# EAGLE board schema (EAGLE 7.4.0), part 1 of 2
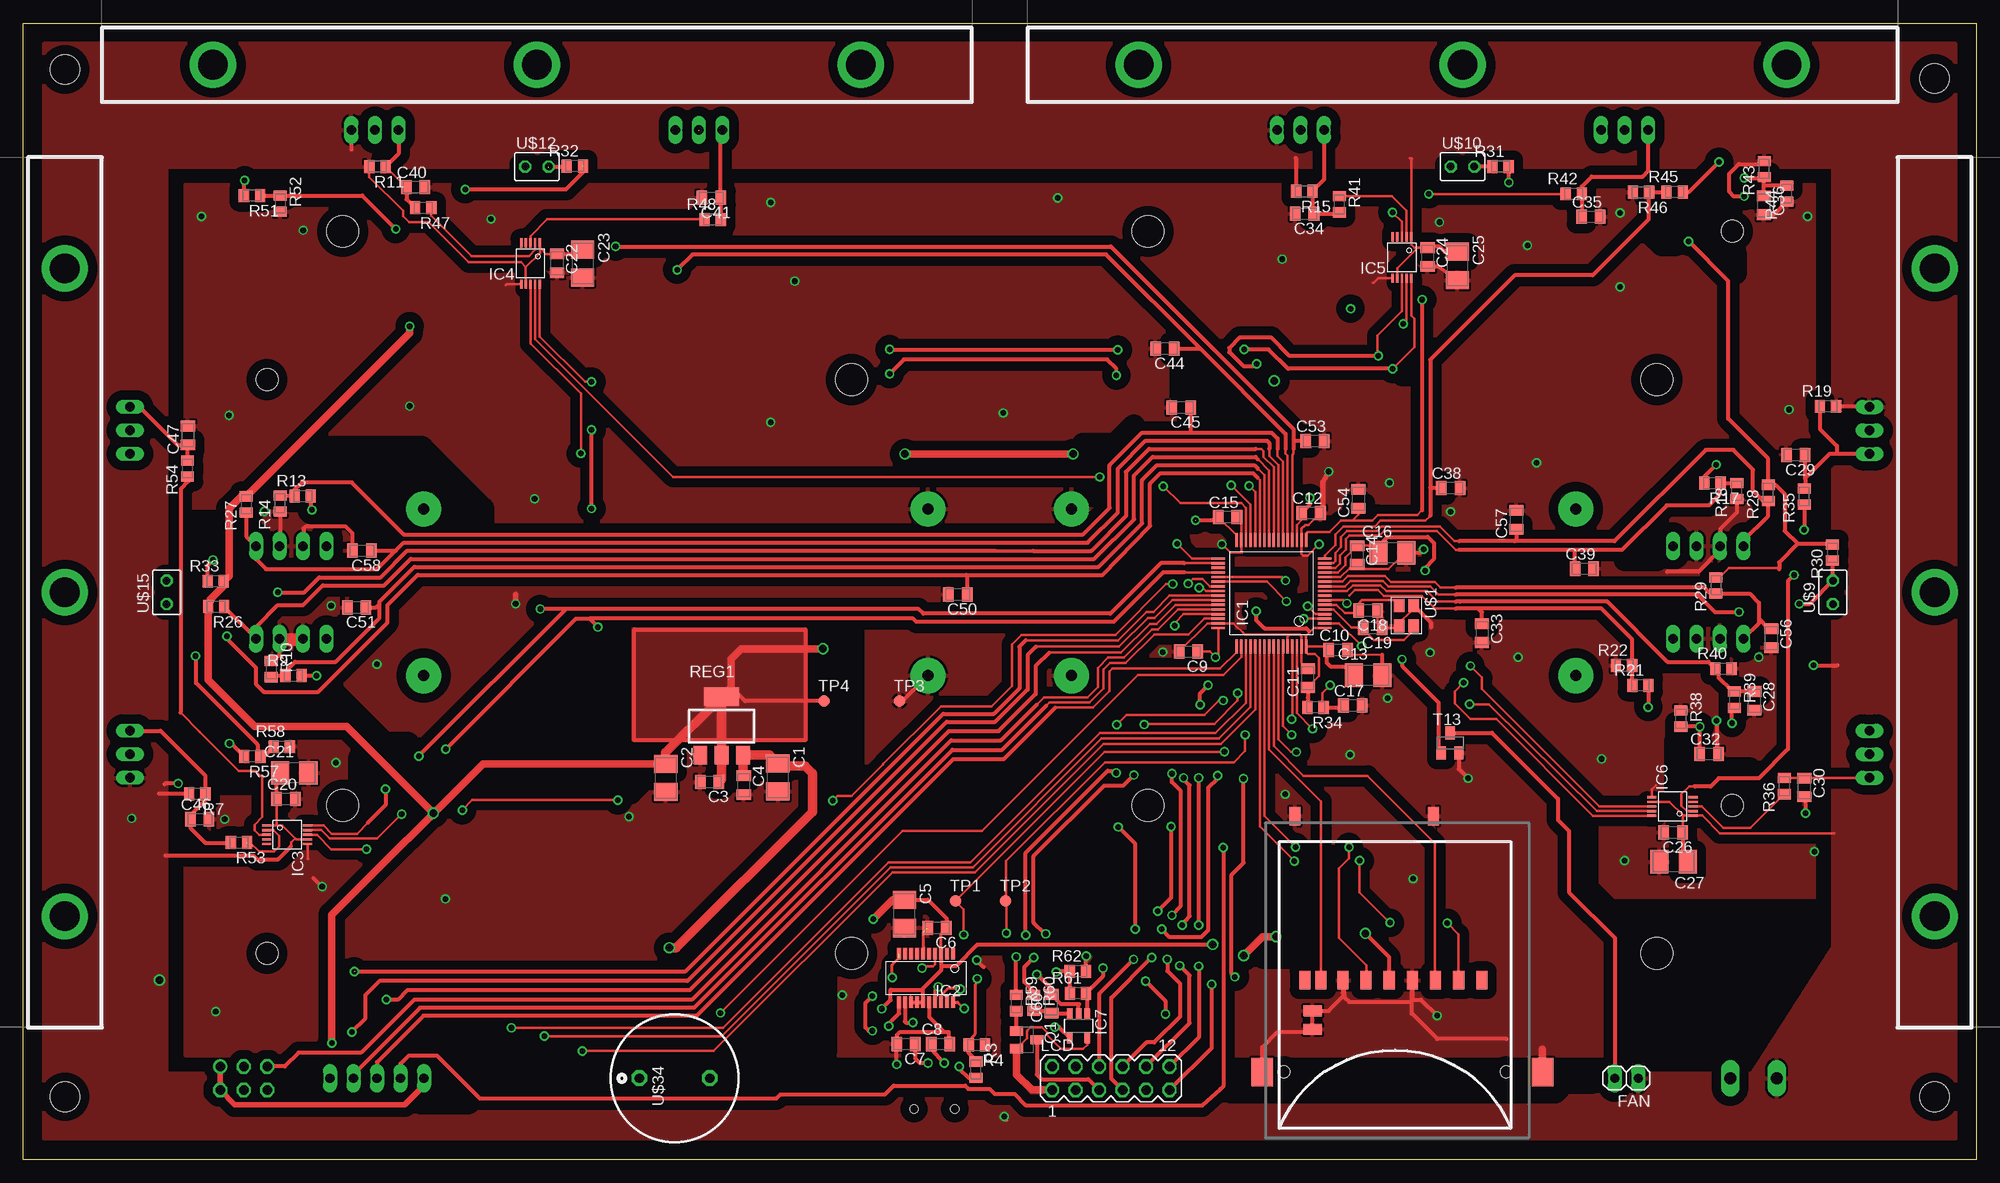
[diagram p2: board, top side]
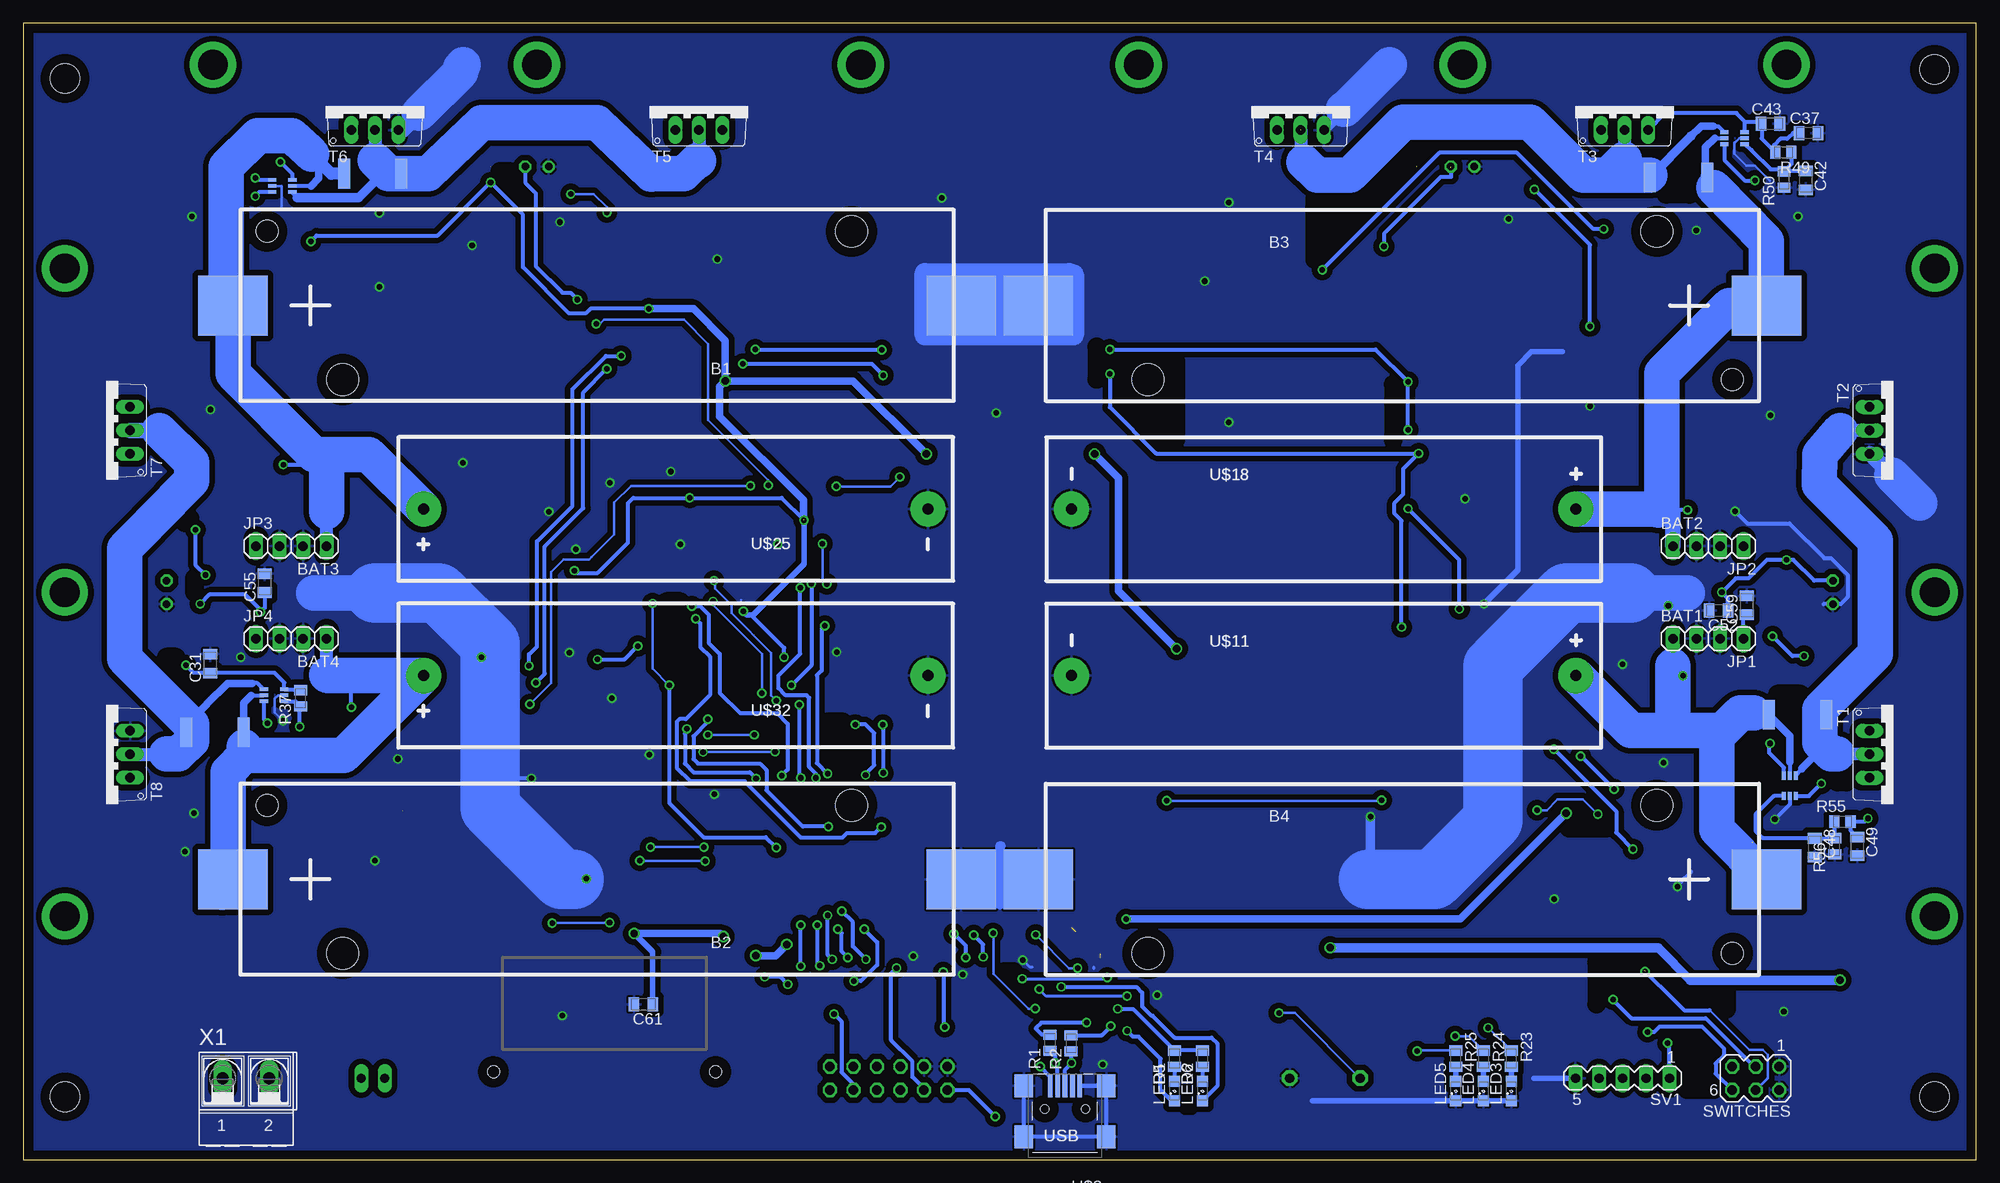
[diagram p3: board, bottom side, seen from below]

Size 211 x 122.79 mm. Coordinates in mm from the lower left corner, seen from the top.
Outline: 0,0 0,122.79 211,122.79 211,0 0,0
Copper layers (1*16): Top 0.035mm / dielectric 1.5mm / Bottom 0.035mm
Design rules "default2": minimum track width 10mil, minimum drill 0.6mm, track to track 8mil, track to pad 8mil, pad to pad 8mil, via to via 8mil, smd to smd 8mil, copper to edge 40mil, drill to drill 8mil, minimum pad ring 10mil, minimum via ring 8mil, stop-mask expansion 4mil, vias tented up to drill 0mil, thermal gap 10mil
Holes 3.2 mm at 4.5,6.79 206.5,6.79 206.5,116.79 4.5,117.79
tRestrict: area 172.2,26.2 to 193.6,27.1; 45 lines
bRestrict: area 51.2,7 to 52.1,7.4; area 54.4,7.2 to 55,7.4; area 84.8,5.4 to 85.5,5.7; area 177.1,110.5 to 177.8,110.7; 19 lines

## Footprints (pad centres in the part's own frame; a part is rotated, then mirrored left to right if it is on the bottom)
KEYSTONE1042 = smd 7.493 x 6.477: P$1 -39.332,0; P$2 39.332,0 | hole 3.454: -27.495,-8.001; 27.495,8.001 | hole 2.388: 35.662,-8.001
1X02 = drill 1.016 long: 1 -1.27,0; 2 1.27,0
SMDB = smd 1.95 x 2.5: P$1 -1.525,0; P$2 1.525,0
SMD0805C = smd 1.143 x 1.524: P$1 -1.016,0; P$2 1.016,0
LQFP64 = smd 0.254 x 1.5: P$1 -3.75,-5.75; P$2 -3.25,-5.75; P$3 -2.75,-5.75; P$4 -2.25,-5.75; P$5 -1.75,-5.75; P$6 -1.25,-5.75; P$7 -0.75,-5.75; P$8 -0.25,-5.75; P$9 0.25,-5.75; P$10 0.75,-5.75; P$11 1.25,-5.75; P$12 1.75,-5.75; P$13 2.25,-5.75; P$14 2.75,-5.75; P$15 3.25,-5.75; P$16 3.75,-5.75; P$33 3.75,5.75; P$34 3.25,5.75; P$35 2.75,5.75; P$36 2.25,5.75; P$37 1.75,5.75; P$38 1.25,5.75; P$39 0.75,5.75; P$40 0.25,5.75; P$41 -0.25,5.75; P$42 -0.75,5.75; P$43 -1.25,5.75; P$44 -1.75,5.75; P$45 -2.25,5.75; P$46 -2.75,5.75; P$47 -3.25,5.75; P$48 -3.75,5.75 | smd 1.5 x 0.254: P$17 5.75,-3.75; P$18 5.75,-3.25; P$19 5.75,-2.75; P$20 5.75,-2.25; P$21 5.75,-1.75; P$22 5.75,-1.25; P$23 5.75,-0.75; P$24 5.75,-0.25; P$25 5.75,0.25; P$26 5.75,0.75; P$27 5.75,1.25; P$28 5.75,1.75; P$29 5.75,2.25; P$30 5.75,2.75; P$31 5.75,3.25; P$32 5.75,3.75; P$49 -5.75,3.75; P$50 -5.75,3.25; P$51 -5.75,2.75; P$52 -5.75,2.25; P$53 -5.75,1.75; P$54 -5.75,1.25; P$55 -5.75,0.75; P$56 -5.75,0.25; P$57 -5.75,-0.25; P$58 -5.75,-0.75; P$59 -5.75,-1.25; P$60 -5.75,-1.75; P$61 -5.75,-2.25; P$62 -5.75,-2.75; P$63 -5.75,-3.25; P$64 -5.75,-3.75
SSOP20 = smd 0.42 x 1.25: P$1 -2.925,-2.625; P$2 -2.275,-2.625; P$3 -1.625,-2.625; P$4 -0.975,-2.625; P$5 -0.325,-2.625; P$6 0.325,-2.625; P$7 0.975,-2.625; P$8 1.625,-2.625; P$9 2.275,-2.625; P$10 2.925,-2.625; P$11 2.925,2.625; P$12 2.275,2.625; P$13 1.625,2.625; P$14 0.975,2.625; P$15 0.325,2.625; P$16 -0.325,2.625; P$17 -0.975,2.625; P$18 -1.625,2.625; P$19 -2.275,2.625; P$20 -2.925,2.625
VSSOP = smd 0.254 x 1: P$1 -1,-2.225; P$2 -0.5,-2.225; P$3 0,-2.225; P$4 0.5,-2.225; P$5 1,-2.225; P$6 1,2.225; P$7 0.5,2.225; P$8 0,2.225; P$9 -0.5,2.225; P$10 -1,2.225
SOT23-5 = smd 0.6 x 1.2: 1 -0.95,-1.306; 2 0,-1.306; 3 0.95,-1.306; 4 0.95,1.306; 5 -0.95,1.306
MA06-2 = drill 1.016 octagon: 1 -6.35,-1.27; 2 -6.35,1.27; 3 -3.81,-1.27; 4 -3.81,1.27; 5 -1.27,-1.27; 6 -1.27,1.27; 7 1.27,-1.27; 8 1.27,1.27; 9 3.81,-1.27; 10 3.81,1.27; 11 6.35,-1.27; 12 6.35,1.27
SML0805 = smd 1.2 x 1.2: A 1.05,0; C -1.05,0
SOT23-BEC = smd 1 x 1.4: B -0.95,-1.1; C 0,1.1; E 0.95,-1.1
SMD0805R = smd 1.1 x 1.4: P$1 -0.875,0; P$2 0.875,0
CURRENT_SENSE = smd 1.3 x 3.2: P$1 -3.1,0; P$2 3.1,0
SOT223 = smd 1.5 x 2: P$1 -2.3,-3.15; P$2 0,-3.15; P$3 2.3,-3.15 | smd 3.8 x 2: P$4 0,3.15
MA05-1 = drill 1.016 long: 1 -5.08,0; 2 -2.54,0; 3 0,0; 4 2.54,0; 5 5.08,0
MA03-2 = drill 1.016: 1 -2.54,-1.27 | drill 1.016 octagon: 2 -2.54,1.27; 3 0,-1.27; 4 0,1.27; 5 2.54,-1.27; 6 2.54,1.27
TO220 = drill 1.016 long: P$1 -2.54,-2.54; P$2 0,-2.54; P$3 2.54,-2.54
SOT23 = smd 1 x 1.4: 1 -0.95,-1.1; 2 0.95,-1.1; 3 0,1.1
B1,27 = smd 1.27 x 1.27: TP 0,0
XTAL-TSX-3225 = smd 1.4 x 1.15: GND1 -1.1,0.8; GND2 1.1,-0.8; P$2 1.1,0.8; P$4 -1.1,-0.8
DCK(INA213) = smd 0.4 x 0.9: P$1 -0.65,-1.1; P$2 0,-1.1; P$3 0.65,-1.1; P$4 0.65,1.1; P$5 0,1.1; P$6 -0.65,1.1
USB-MINI = smd 2 x 2.5: M1 -4.45,-2.25; M2 4.45,-2.25; M3 -4.45,-7.75; M4 4.45,-7.75 | smd 0.5 x 2.5: P$1 1.6,-7.75; P$2 0.8,-7.75; P$3 0,-7.75; P$4 -0.8,-7.75; P$5 -1.6,-7.75 | hole 0.9: -2.2,-5.25; 2.2,-5.25
THERMISTOR = drill 0.813 octagon: 1 -1.27,0; 2 1.27,0
KEYSTONE1015 = drill 1.2 pad 3.81: P$1 -27.241,0; P$2 27.241,0
CHLADIC = drill 3.2 pad 5: P$1 -35,23.5; P$2 0,23.5; P$4 35,23.5
SD-SOCKET = smd 1.2 x 2: DC -10.83,17.75; OPT 4.15,17.75; P$1 6.87,0; P$2 4.37,0; P$3 1.87,0; P$4 -0.63,0; P$5 -3.13,0; P$6 -5.63,0; P$7 -8,0; P$8 -9.75,0; P$9 9.37,0 | smd 2 x 1.2: GND -8.9,-3.3; WP -8.9,-5.3 | smd 2.3 x 3.1: M1 15.95,-9.9; M2 -14.35,-9.9 | hole 1.3: 12,-9.9; -12,-9.9
12N40 = drill 1 pad 1.676 octagon: P$1 0,3.8; P$2 0,-3.8
AK500/2-H = drill 1.321 long: 1 -2.515,0; 2 2.515,0

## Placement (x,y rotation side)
B1  BATTERY-LI  [KEYSTONE1042]  149,92.29 180 bottom
B2  BATTERY-LI  [KEYSTONE1042]  149,30.29 180 bottom
B3  BATTERY-LI  [KEYSTONE1042]  62,92.29 0 bottom
B4  BATTERY-LI  [KEYSTONE1042]  62,30.29 0 bottom
BAT1  [1X02]  31.5,56.29 0 bottom
BAT2  [1X02]  31.5,66.29 0 bottom
BAT3  [1X02]  179.5,66.29 180 bottom
BAT4  [1X02]  179.5,56.29 180 bottom
C1  10uF  [SMDB]  81.53,41.29 270 top
C2  10uF  [SMDB]  69.42,41.24 270 top
C3  100n  [SMD0805C]  74.15,40.81 180 top
C4  100n  [SMD0805C]  77.85,40.46 270 top
C5  4.7uF  [SMDB]  95.2,26.54 270 top
C6  100n  [SMD0805C]  98.72,25.04 180 top
C7  47pF  [SMD0805C]  95.38,12.49 180 top
C8  47pF  [SMD0805C]  99.1,12.49 0 top
C9  100n  [SMD0805C]  125.88,54.88 180 top
C10  100n  [SMD0805C]  142.07,55.06 0 top
C11  100n  [SMD0805C]  138.77,52.02 90 top
C12  100n  [SMD0805C]  139.13,69.87 0 top
C13  10uF  [SMDB]  145.3,52.33 0 top
C14  100n  [SMD0805C]  144.11,65.31 270 top
C15  100n  [SMD0805C]  130.11,69.41 0 top
C16  1uF  [SMDB]  147.91,65.57 0 top
C17  100n  [SMD0805C]  143.64,49.06 0 top
C18  25pF  [SMD0805C]  145.3,59.34 180 top
C19  25pF  [SMD0805C]  145.77,57.44 180 top
C20  100n  [SMD0805C]  28.39,38.96 0 top
C21  10uF  [SMDB]  29.3,41.79 0 top
C22  100n  [SMD0805C]  57.67,96.83 270 top
C23  10uF  [SMDB]  60.45,96.81 270 top
C24  100n  [SMD0805C]  151.72,97.51 270 top
C25  10uF  [SMDB]  154.93,96.55 270 top
C26  100n  [SMD0805C]  178.25,35.34 180 top
C27  10uF  [SMDB]  178.3,32.19 180 top
C28  100n  [SMD0805C]  187,49.56 270 top
C29  22n  [SMD0805C]  191.5,76.11 180 top
C30  22n  [SMD0805C]  192.43,40.21 270 top
C31  100n  [SMD0805C]  190.8,53.59 90 bottom
C32  100n  [SMD0805C]  182.12,43.84 0 top
C33  100n  [SMD0805C]  157.6,56.89 270 top
C34  22n  [SMD0805C]  138.43,102.19 180 top
C35  22n  [SMD0805C]  169.35,101.86 0 top
C36  100n  [SMD0805C]  188.05,103.11 270 top
C37  100n  [SMD0805C]  18.12,110.91 0 bottom
C38  100n  [SMD0805C]  154.2,72.56 0 top
C39  100n  [SMD0805C]  168.65,63.84 0 top
C40  22n  [SMD0805C]  42.4,105.06 0 top
C41  22n  [SMD0805C]  74.35,103.91 180 top
C42  100n  [SMD0805C]  18.42,105.79 270 bottom
C43  100n  [SMD0805C]  22.25,111.91 0 bottom
C44  100n  [SMD0805C]  123.35,87.61 180 top
C45  100n  [SMD0805C]  125.1,81.26 180 top
C46  22n  [SMD0805C]  19.08,36.79 0 top
C47  22n  [SMD0805C]  17.8,78.24 90 top
C48  100n  [SMD0805C]  17.45,33.69 270 bottom
C49  100n  [SMD0805C]  12.88,33.84 270 bottom
C50  100n  [SMD0805C]  100.97,61.06 180 top
C51  100n  [SMD0805C]  36.03,59.66 180 top
C52  100n  [SMD0805C]  27.85,59.34 180 bottom
C53  100n  [SMD0805C]  139.55,77.64 0 top
C54  100n  [SMD0805C]  144.25,71.39 90 top
C55  100n  [SMD0805C]  184.9,62.29 90 bottom
C56  100n  [SMD0805C]  188.85,56.34 270 top
C57  100n  [SMD0805C]  161.3,69.14 90 top
C58  100n  [SMD0805C]  36.6,65.79 180 top
C59  100n  [SMD0805C]  24.8,59.89 90 bottom
C60  100n  [SMD0805C]  111.07,16.84 90 top
C61  100n  [SMD0805C]  144,16.79 180 bottom
FAN  [1X02]  173.21,8.79 180 top
IC1  [LQFP64]  134.85,61.19 90 top
IC2  FT231XS  [SSOP20]  97.53,19.63 180 top
IC3  DAC122S085  [VSSOP]  28.52,35.1 270 top
IC4  DAC122S085  [VSSOP]  54.8,96.81 180 top
IC5  DAC122S085  [VSSOP]  148.94,97.46 180 top
IC6  DAC122S085  [VSSOP]  178.18,38.15 90 top
IC7  MCP601OT  [SOT23-5]  114.02,14.45 180 top
JP1  TH1  [1X02]  26.42,56.29 180 bottom
JP2  TH2  [1X02]  26.42,66.29 180 bottom
JP3  TH3  [1X02]  184.58,66.29 0 bottom
JP4  TH4  [1X02]  184.58,56.29 0 bottom
LCD  [MA06-2]  117.5,8.79 0 top
LED1  G  [SML0805]  86.62,7.41 90 bottom
LED2  R  [SML0805]  83.6,7.41 90 bottom
LED3  [SML0805]  50.25,7.41 90 bottom
LED4  [SML0805]  53.25,7.41 90 bottom
LED5  [SML0805]  56.25,7.41 90 bottom
Q1  BC807-16LT1SMD  [SOT23-BEC]  108.42,12.95 270 top
R1  27  [SMD0805R]  100.08,12.61 90 bottom
R2  27  [SMD0805R]  97.8,12.56 90 bottom
R3  4k7  [SMD0805R]  102.92,9.71 270 top
R4  10k  [SMD0805R]  103.03,12.39 180 top
R5  270  [SMD0805R]  86.62,10.91 90 bottom
R6  270  [SMD0805R]  83.6,10.91 90 bottom
R7  33k  [SMD0805R]  18.83,39.51 180 top
R8  33m  [CURRENT_SENSE]  19.33,48.05 180 bottom
R9  100k  [SMD0805R]  29.2,52.29 0 top
R10  56k  [SMD0805R]  26.8,52.99 270 top
R11  33k  [SMD0805R]  38.28,107.29 180 top
R12  33m  [CURRENT_SENSE]  32.18,106.11 0 bottom
R13  100k  [SMD0805R]  30.2,71.69 0 top
R14  56k  [SMD0805R]  27.75,70.89 90 top
R15  33k  [SMD0805R]  138.4,104.61 180 top
R16  33m  [CURRENT_SENSE]  173.25,106.52 180 bottom
R17  100k  [SMD0805R]  182.5,73.09 180 top
R18  56k  [SMD0805R]  185.1,72.24 90 top
R19  33k  [SMD0805R]  194.97,81.39 0 top
R20  33m  [CURRENT_SENSE]  190.28,46.16 0 bottom
R21  100k  [SMD0805R]  174.7,51.24 0 top
R22  56k  [SMD0805R]  172.93,53.39 0 top
R23  270  [SMD0805R]  50.25,10.91 270 bottom
R24  270  [SMD0805R]  53.25,10.91 270 bottom
R25  270  [SMD0805R]  56.25,10.91 270 bottom
R26  33k  [SMD0805R]  20.85,59.74 180 top
R27  33k  [SMD0805R]  24.1,70.79 90 top
R28  33k  [SMD0805R]  188.5,72.04 90 top
R29  33k  [SMD0805R]  182.88,62.03 90 top
R30  33k  [SMD0805R]  195.45,65.59 90 top
R31  33k  [SMD0805R]  159.6,107.29 0 top
R32  33k  [SMD0805R]  59.6,107.34 0 top
R33  33k  [SMD0805R]  20.8,62.49 0 top
R34  10k  [SMD0805R]  139.62,48.86 180 top
R35  10R  [SMD0805R]  192.4,71.64 90 top
R36  10R  [SMD0805R]  190.25,40.36 90 top
R37  10k  [SMD0805R]  181.03,49.84 90 bottom
R38  10k  [SMD0805R]  179.07,47.64 270 top
R39  5k6  [SMD0805R]  184.88,49.69 270 top
R40  10k  [SMD0805R]  183.68,53.04 0 top
R41  10R  [SMD0805R]  142.18,103.21 270 top
R42  10R  [SMD0805R]  167.5,104.34 0 top
R43  10k  [SMD0805R]  188.07,107.01 90 top
R44  10k  [SMD0805R]  190.5,104.36 90 top
R45  5k6  [SMD0805R]  178.4,104.54 0 top
R46  10k  [SMD0805R]  174.78,104.51 180 top
R47  10R  [SMD0805R]  43.23,102.84 180 top
R48  10R  [SMD0805R]  74.5,101.56 0 top
R49  10k  [SMD0805R]  20.85,108.84 180 bottom
R50  10k  [SMD0805R]  20.78,105.89 90 bottom
R51  5k6  [SMD0805R]  24.72,104.16 180 top
R52  10k  [SMD0805R]  27.78,103.29 270 top
R53  10R  [SMD0805R]  23.33,34.26 180 top
R54  10R  [SMD0805R]  17.75,74.66 90 top
R55  10k  [SMD0805R]  14.47,36.51 0 bottom
R56  10k  [SMD0805R]  15.3,33.86 90 bottom
R57  5k6  [SMD0805R]  24.75,43.56 180 top
R58  10k  [SMD0805R]  27.95,44.61 0 top
R59  33k  [SMD0805R]  107.28,16.92 270 top
R60  33k  [SMD0805R]  109.17,16.94 270 top
R61  33k  [SMD0805R]  113.95,17.97 0 top
R62  33k  [SMD0805R]  113.93,20.35 0 top
REG1  NCP1117ST33T3G  [SOT223]  75.45,46.84 0 top
SV1  SWD  [MA05-1]  38.23,8.79 180 bottom
SWITCHES  [MA03-2]  23.83,8.79 180 bottom
T1  NDP6020P  [TO220]  9,43.79 270 bottom
T2  STP80NF03L-04  [TO220]  9,78.79 270 bottom
T3  NDP6020P  [TO220]  38,113.79 0 bottom
T4  STP80NF03L-04  [TO220]  73,113.79 0 bottom
T5  NDP6020P  [TO220]  138,113.79 0 bottom
T6  STP80NF03L-04  [TO220]  173,113.79 0 bottom
T7  NDP6020P  [TO220]  202,78.79 90 bottom
T8  STP80NF03L-04  [TO220]  202,43.79 90 bottom
T13  2N7002  [SOT23]  154.15,45.02 0 top
TP1  PTR1B1,27  [B1,27]  100.7,27.94 0 top
TP2  PTR1B1,27  [B1,27]  106.1,27.94 0 top
TP3  PTR1B1,27  [B1,27]  94.65,49.54 0 top
TP4  PTR1B1,27  [B1,27]  86.5,49.54 0 top
U$1  XTAL  [XTAL-TSX-3225]  149.43,58.77 270 top
U$2  INA213A  [DCK(INA213)]  183.9,50.16 90 bottom
U$3  USB-MINI  [USB-MINI]  98.45,0.22 180 bottom
U$4  INA213A  [DCK(INA213)]  183,105.19 270 bottom
U$5  INA213A  [DCK(INA213)]  26.12,110.36 90 bottom
U$6  INA213A  [DCK(INA213)]  20.15,40.39 0 bottom
U$9  THERMISTOR  [THERMISTOR]  195.5,61.29 90 top
U$10  THERMISTOR  [THERMISTOR]  155.5,107.29 0 top
U$11  BATTERY-AA  [KEYSTONE1015]  70.5,52.29 0 bottom
U$12  THERMISTOR  [THERMISTOR]  55.5,107.29 0 top
U$15  THERMISTOR  [THERMISTOR]  15.5,61.29 90 top
U$16  CHLADIC  [CHLADIC]  230,61.29 90 top
U$17  CHLADIC  [CHLADIC]  -19,61.29 270 top
U$18  BATTERY-AA  [KEYSTONE1015]  70.5,70.29 0 bottom
U$19  CHLADIC  [CHLADIC]  55.5,141.79 180 top
U$22  CHLADIC  [CHLADIC]  155.5,141.79 180 top
U$25  BATTERY-AA  [KEYSTONE1015]  140.5,70.29 180 bottom
U$32  BATTERY-AA  [KEYSTONE1015]  140.5,52.29 180 bottom
U$33  SD-CARD  [SD-SOCKET]  148.2,19.37 0 top
U$34  12N40  [12N40]  70.38,8.79 90 top
X1  [AK500/2-H]  186.93,8.79 0 bottom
